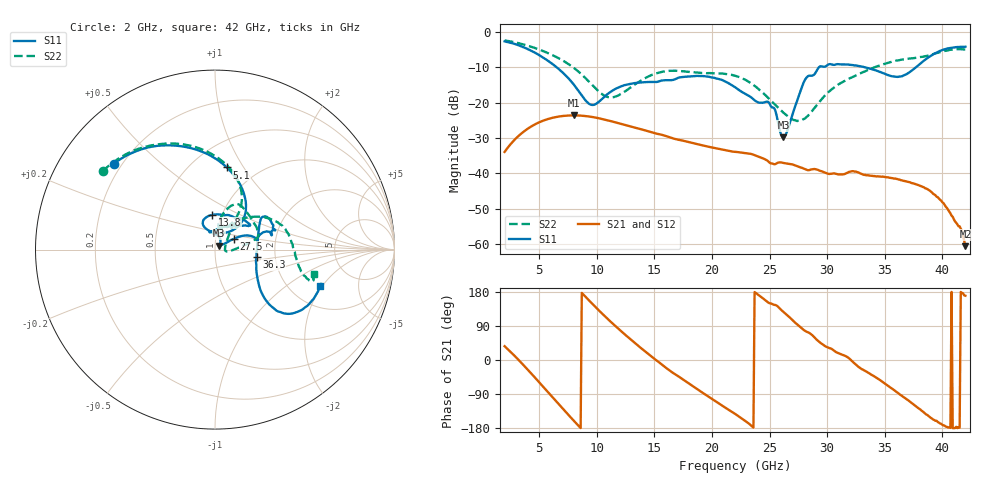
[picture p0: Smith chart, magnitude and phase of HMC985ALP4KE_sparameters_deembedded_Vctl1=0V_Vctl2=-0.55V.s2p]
!s2p File: Measurements: S11, S21, S12, S22
# GHz S dB R 50.0
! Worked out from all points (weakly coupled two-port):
!   401 points, 2 GHz to 42 GHz, reference 50 ohm
!   highest |S21| = -23.58 dB at 8 GHz (marker M1); lowest = -60.6 dB at 42 GHz (marker M2)
!   lowest |S11| = -29.8 dB at 26.2 GHz (marker M3), VSWR 1.07, Z = 52.4 + j2.23 ohm
!   |S11| at or under -10 dB: 6.536 GHz to 29.27 GHz (22.74 GHz wide, 127 % of centre); 33.34 GHz to 37.69 GHz (4.347 GHz wide, 12.2 % of centre)
!   |S22| runs from -25.2 to -2.3 dB; largest |S21 - S12| = 0.00022
!   S11 on the Smith chart (normalised r, x): 2 GHz: 0.17, +0.36; 5.1 GHz: 0.73, +0.85; 13.8 GHz: 0.90, +0.36; 27.5 GHz: 1.22, +0.15; 36.3 GHz: 1.59, -0.14; 42 GHz: 2.91, -1.91
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2  -2.61 139.7  -33.94 36.4  -33.94 36.3  -2.35 145.1
3.5  -4.08 111.8  -28.60 -9.0  -28.60 -9.0  -3.36 121.1
5.1  -6.70 81.8  -25.40 -62.1  -25.41 -62.1  -5.05 96.7
8  -14.83 45.2  -23.58 -160.1  -23.59 -160.1  -10.10 61.4
8.7  -17.96 51.6  -23.68 177.1  -23.68 177.1  -12.03 57.4
9.7  -20.62 86.6  -24.09 145.6  -24.09 145.6  -15.29 57.7
11.1  -17.13 115.4  -25.11 104.0  -25.11 104.0  -18.47 73.0
13.8  -14.26 95.3  -27.48 32.4  -27.48 32.4  -13.78 77.2
15.4  -13.94 73.0  -28.90 -5.9  -28.90 -6.0  -11.44 68.3
19.4  -12.52 34.7  -32.24 -90.7  -32.25 -90.7  -11.59 35.1
22  -15.59 52.2  -33.91 -142.0  -33.92 -142.1  -12.35 15.1
25  -20.22 97.7  -36.97 149.9  -36.99 149.7  -19.04 1.3
26.2  -29.81 41.1  -37.04 126.9  -37.06 126.8  -22.81 -8.3
27.5  -18.42 29.6  -38.10 91.1  -38.10 90.8  -25.09 1.8
28.1  -13.37 20.7  -38.84 76.5  -38.87 76.5  -24.37 18.4
28.7  -12.32 12.8  -38.85 65.7  -38.87 65.6  -22.31 33.1
31  -9.09 23.4  -40.32 17.7  -40.29 17.9  -14.77 52.8
35.4  -12.27 12.4  -41.24 -70.9  -41.23 -70.5  -8.59 25.1
36.3  -12.57 -10.2  -41.80 -90.8  -41.80 -90.4  -7.91 17.6
39.7  -5.45 -42.0  -47.15 -165.3  -47.19 -166.0  -5.76 -16.2
41.5  -4.18 -23.0  -55.03 -178.7  -55.33 -177.6  -4.80 -17.1
42  -4.14 -19.0  -60.65 169.6  -59.88 174.7  -4.94 -14.2
